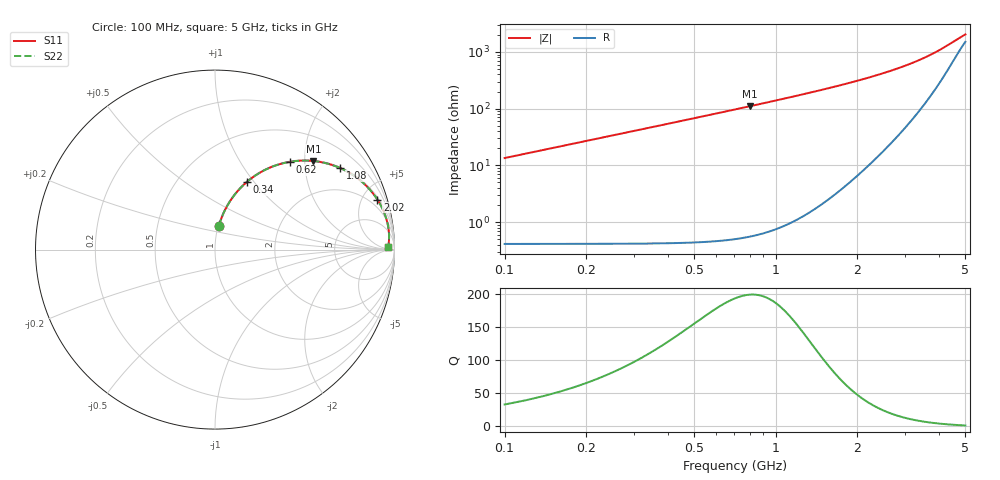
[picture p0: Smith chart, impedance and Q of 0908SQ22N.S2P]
! Coilcraft 0908SQ-22N Air Core Inductor
! 07 March 2008
# MHZ S MA R 50
!Freq  MagS11  AngS11  MagS21  AngS21  MagS12  AngS12  MagS22  AngS22
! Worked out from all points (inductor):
!   246 points, 100 MHz to 5 GHz, reference 50 ohm
!   read as one part in series: L = 21.4 nH near 120 MHz
!   highest Q = 199 at 800 MHz (marker M1), where L = 21.9 nH
!   S11 on the Smith chart (normalised r, x): 100 MHz: 1.01, +0.27; 340 MHz: 1.01, +0.92; 620 MHz: 1.01, +1.69; 1.08 GHz: 1.03, +3.04; 2.02 GHz: 1.20, +6.44; 5 GHz: 49, +17
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100  0.1326 80.6  0.9871 -7.6  0.9871 -7.6  0.1326 80.6
120  0.1586 79.4  0.9833 -9.1  0.9833 -9.1  0.1586 79.4
140  0.1842 78.1  0.9789 -10.6  0.9789 -10.6  0.1842 78.1
160  0.2094 76.8  0.9738 -12.1  0.9738 -12.1  0.2094 76.8
200  0.2587 74.1  0.962 -15.0  0.962 -15.0  0.2587 74.1
260  0.3291 70.1  0.9404 -19.3  0.9404 -19.3  0.3291 70.1
340  0.4152 64.9  0.9059 -24.6  0.9059 -24.6  0.4152 64.9
460  0.5266 57.7  0.8465 -31.9  0.8465 -31.9  0.5266 57.7
540  0.5891 53.4  0.8045 -36.2  0.8045 -36.2  0.5892 53.4
620  0.643 49.5  0.7623 -40.2  0.7623 -40.2  0.643 49.5
800  0.7375 42.0  0.6716 -47.7  0.6716 -47.7  0.7375 42.0
920  0.7842 37.9  0.6165 -51.8  0.6165 -51.8  0.7842 37.9
1080  0.8315 33.2  0.5507 -56.5  0.5507 -56.5  0.8316 33.2
1220  0.8627 29.7  0.5 -59.9  0.5 -59.9  0.8627 29.7
1380  0.8897 26.4  0.4492 -63.1  0.4492 -63.1  0.8897 26.4
1740  0.929 20.5  0.357 -68.6  0.357 -68.6  0.929 20.5
2020  0.9469 17.1  0.3013 -71.7  0.3013 -71.7  0.947 17.1
2560  0.9654 12.1  0.2198 -75.2  0.2198 -75.2  0.9654 12.1
3380  0.9737 7.0  0.1354 -75.7  0.1354 -75.7  0.9737 7.0
4200  0.9714 3.4  0.07938 -67.7  0.07938 -67.7  0.9714 3.4
4720  0.9671 1.6  0.05569 -53.5  0.05569 -53.5  0.9671 1.6
5000  0.9642 0.7  0.0475 -41.3  0.0475 -41.3  0.9642 0.7
